FUNCTION_BLOCK "Main"
VERSION : 0.1
   VAR_TEMP
      temp1 : Bool;
   END_VAR


BEGIN
NETWORK
TITLE =
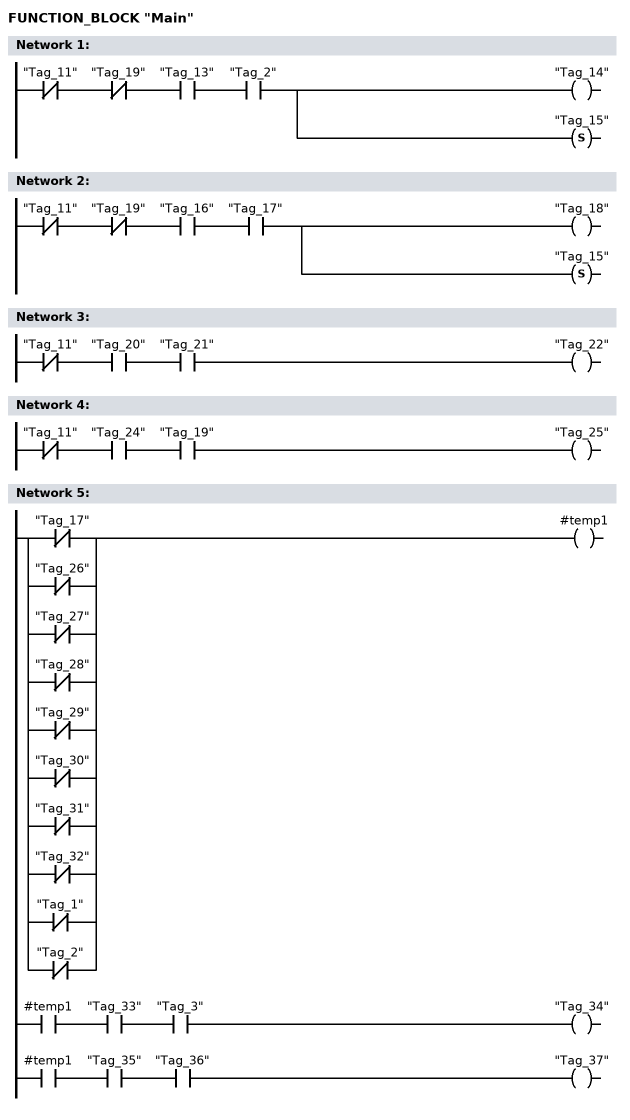
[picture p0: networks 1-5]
      AN "Tag_11";
      AN "Tag_19";
      A "Tag_13";
      A "Tag_2";
      = "Tag_14";
      S "Tag_15";
NETWORK
TITLE =
      AN "Tag_11";
      AN "Tag_19";
      A "Tag_16";
      A "Tag_17";
      = "Tag_18";
      S "Tag_15";
NETWORK
TITLE =
      AN "Tag_11";
      A "Tag_20";
      A "Tag_21";
      = "Tag_22";
NETWORK
TITLE =
      AN "Tag_11";
      A "Tag_24";
      A "Tag_19";
      = "Tag_25";
NETWORK
TITLE =
      A(;
      ON "Tag_17";
      ON "Tag_26";
      ON "Tag_27";
      ON "Tag_28";
      ON "Tag_29";
      ON "Tag_30";
      ON "Tag_31";
      ON "Tag_32";
      ON "Tag_1";
      ON "Tag_2";
      );
      = #temp1;
      A #temp1;
      A "Tag_33";
      A "Tag_3";
      = "Tag_34";
      A #temp1;
      A "Tag_35";
      A "Tag_36";
      = "Tag_37";
END_FUNCTION_BLOCK

TAG
"Tag_1","%I0.0","Bool","True","True","False","","","True"
"Tag_2","%I0.1","Bool","True","True","False","","","True"
"Tag_3","%I0.2","Bool","True","True","False","","","True"
"Tag_5","%I5.0","Bool","True","True","False","","","True"
"Tag_6","%I5.1","Bool","True","True","False","","","True"
"Tag_7","%Q0.1","Bool","True","True","False","","","True"
"Tag_8","%I2.1","Bool","True","True","False","","","True"
"Tag_11","%I0.3","Bool","True","True","False","","","True"
"Tag_12","%I3.0","Bool","True","True","False","","","True"
"Tag_13","%I5.5","Bool","True","True","False","","","True"
"Tag_14","%Q1.0","Bool","True","True","False","","","True"
"Tag_15","%Q1.2","Bool","True","True","False","","","True"
"Tag_16","%I5.4","Bool","True","True","False","","","True"
"Tag_17","%I1.0","Bool","True","True","False","","","True"
"Tag_18","%Q1.1","Bool","True","True","False","","","True"
"Tag_19","%I3.6","Bool","True","True","False","","","True"
"Tag_20","%I5.3","Bool","True","True","False","","","True"
"Tag_21","%I0.5","Bool","True","True","False","","","True"
"Tag_22","%Q1.5","Bool","True","True","False","","","True"
"Tag_23","%I3.3","Bool","True","True","False","","","True"
"Tag_24","%I5.6","Bool","True","True","False","","","True"
"Tag_25","%Q1.6","Bool","True","True","False","","","True"
"Tag_26","%I1.1","Bool","True","True","False","","","True"
"Tag_27","%I1.2","Bool","True","True","False","","","True"
"Tag_28","%I1.3","Bool","True","True","False","","","True"
"Tag_29","%I1.4","Bool","True","True","False","","","True"
"Tag_30","%I1.5","Bool","True","True","False","","","True"
"Tag_31","%I1.6","Bool","True","True","False","","","True"
"Tag_32","%I1.7","Bool","True","True","False","","","True"
"Tag_33","%I5.7","Bool","True","True","False","","","True"
"Tag_34","%Q1.3","Bool","True","True","False","","","True"
"Tag_35","%I4.0","Bool","True","True","False","","","True"
"Tag_36","%I0.4","Bool","True","True","False","","","True"
"Tag_37","%Q1.4","Bool","True","True","False","","","True"
"Tag_38","%I2.0","Bool","True","True","False","","","True"
"Tag_39","%I3.7","Bool","True","True","False","","","True"
"Tag_40","%I2.3","Bool","True","True","False","","","True"
"Tag_41","%Q0.3","Bool","True","True","False","","","True"
"Tag_42","%Q0.0","Bool","True","True","False","","","True"
"Tag_43","%I2.2","Bool","True","True","False","","","True"
"Tag_44","%I3.5","Bool","True","True","False","","","True"
"Tag_45","%I5.2","Bool","True","True","False","","","True"
"Tag_46","%M1.0","Bool","True","True","False","","","True"
END_TAG
